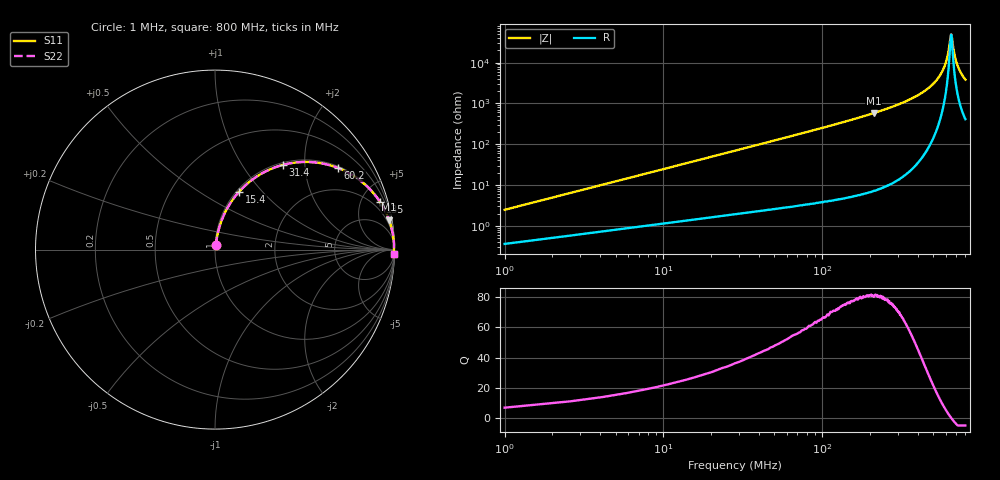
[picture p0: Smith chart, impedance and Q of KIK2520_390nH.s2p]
!version-2
!date-01.2022
!Series
# MHz S RI R 50
!Freq ReS11 ImS11 ReS21 ImS21 ReS12 ImS12 ReS22 ImS22
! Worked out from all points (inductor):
!   501 points, 1 MHz to 800 MHz, reference 50 ohm
!   read as one part in series: L = 390 nH near 4.2 MHz
!   highest Q = 81.3 at 212 MHz (marker M1), where L = 437 nH
!   self-resonance near 651 MHz
!   S11 on the Smith chart (normalised r, x): 1 MHz: 1.01, +0.05; 15.4 MHz: 1.03, +0.76; 31.4 MHz: 1.04, +1.54; 60.2 MHz: 1.06, +2.98; 135 MHz: 1.09, +6.93; 800 MHz: 9, -76
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1  0.00418 0.0243  0.9958 -0.0243  0.9958 -0.0243  0.00418 0.0243
5.8  0.0279 0.137  0.9721 -0.137  0.9721 -0.137  0.0279 0.137
7.4  0.0406 0.1723  0.9594 -0.1723  0.9594 -0.1723  0.0406 0.1723
15.4  0.134 0.3224  0.866 -0.3224  0.866 -0.3224  0.134 0.3224
31.4  0.3763 0.4715  0.6237 -0.4715  0.6237 -0.4715  0.3763 0.4715
60.2  0.6856 0.4548  0.3144 -0.4548  0.3144 -0.4548  0.6856 0.4548
90.6  0.8329 0.3653  0.1671 -0.3653  0.1671 -0.3653  0.8329 0.3653
135  0.9202 0.2643  0.0798 -0.2643  0.0798 -0.2643  0.9202 0.2643
212  0.9694 0.1662  0.0306 -0.1662  0.0306 -0.1662  0.9694 0.1662
268  0.9827 0.1239  0.0173 -0.1239  0.0173 -0.1239  0.9827 0.1239
401  0.9947 0.0627  0.00534 -0.0627  0.00534 -0.0627  0.9947 0.0627
534  0.9978 0.025  0.00224 -0.025  0.00224 -0.025  0.9978 0.025
571  0.998 0.0165  0.002 -0.0165  0.002 -0.0165  0.998 0.0165
603  0.9981 0.00969  0.00194 -0.00969  0.00194 -0.00969  0.9981 0.00969
627  0.998 0.00481  0.00196 -0.00481  0.00196 -0.00481  0.998 0.00481
649  0.998 0.000425  0.00203 -0.000425  0.00203 -0.000425  0.998 0.000425
654  0.9979 -0.000494  0.00205 0.000494  0.00205 0.000494  0.9979 -0.000494
667  0.9979 -0.00291  0.00212 0.00291  0.00212 0.00291  0.9979 -0.00291
687  0.9978 -0.00675  0.00225 0.00675  0.00225 0.00675  0.9978 -0.00675
711  0.9976 -0.011  0.00244 0.011  0.00244 0.011  0.9976 -0.011
751  0.9972 -0.0179  0.00285 0.0179  0.00285 0.0179  0.9972 -0.0179
800  0.9965 -0.0258  0.00346 0.0258  0.00346 0.0258  0.9965 -0.0258
